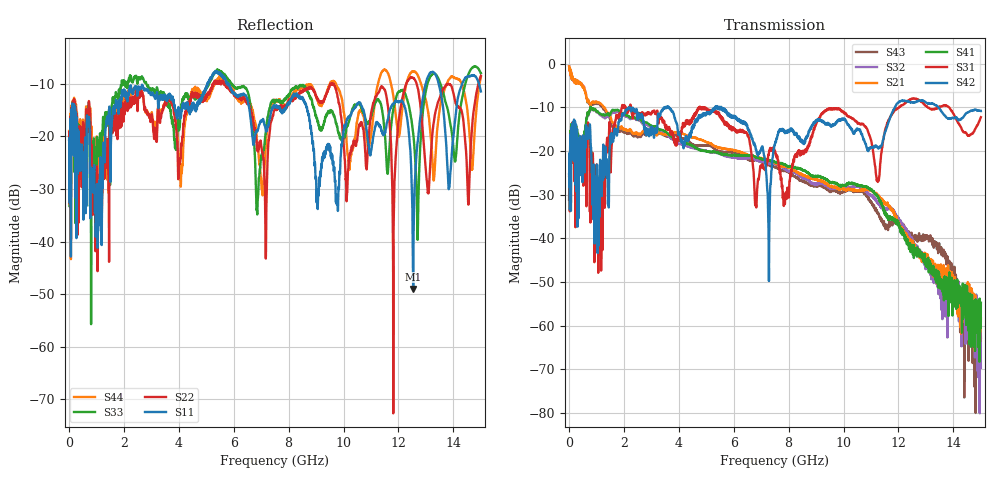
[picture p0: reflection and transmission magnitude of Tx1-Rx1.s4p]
! FILE: N:\QM 2007\Prüfprotokolle\Highspeed\Konfektionierte Ltg\L45593-D106\D30\8216\0002  kpl\IL  mit Chris Boards\Tx1-Rx1.s4p
# MHz S DB R 50.00
! FREQ  S11  S12  S13  S14
!  S21  S22  S23  S24
!  S31  S32  S33  S34
!  S41  S42  S43  S44
!  DB  ANG  DB  ANG  DB  ANG  DB  ANG
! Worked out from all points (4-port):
!   2999 points, 10 MHz to 15 GHz, reference 50 ohm
!   strongest paths, dB at 10 MHz, 3.755 GHz, 7.505 GHz, 11.26 GHz, 15 GHz:
!     S42: -25.1, -10.8, -18.3, -19.1, -10.9
!     S31: -25.7, -15.5, -20.1, -26.8, -12.3
!     S41: -31.1, -16.8, -22.5, -30.5, -54.7
!     S21: -0.6, -15.9, -22.8, -30.2, -58.4
!     S32: -31.3, -17.2, -22.9, -32.0, -69.6
!     S43: -0.6, -16.5, -23.7, -34.2, -62.8
!   lowest |S11| = -49.0 dB at 12.54 GHz (marker M1), VSWR 1.01, Z = 50.1 - j0.325 ohm
!   |S11| at or under -10 dB: start of sweep to 5.039 GHz; 5.813 GHz to 12.99 GHz (7.178 GHz wide, 76.3 % of centre); 13.46 GHz to 14.32 GHz (855.5 MHz wide, 6.16 % of centre)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
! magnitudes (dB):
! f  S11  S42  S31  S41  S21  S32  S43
! 10 MHz  -20.6  -25.1  -25.7  -31.1  -0.6  -31.3  -0.6
! 11.4 GHz  -19.2  -18.4  -19.2  -32.5  -31.0  -33.1  -35.9
! 11.82 GHz  -13.8  -10.5  -11.1  -35.9  -33.8  -33.5  -36.5
! 12.54 GHz  -49.0  -8.9  -7.9  -42.3  -41.4  -41.2  -39.9
! 13.11 GHz  -8.3  -9.0  -10.1  -47.8  -45.2  -46.3  -40.4
! 13.85 GHz  -29.7  -12.7  -10.0  -52.7  -48.8  -51.0  -45.6
! 15 GHz  -11.5  -10.9  -12.3  -54.7  -58.4  -69.6  -62.8
